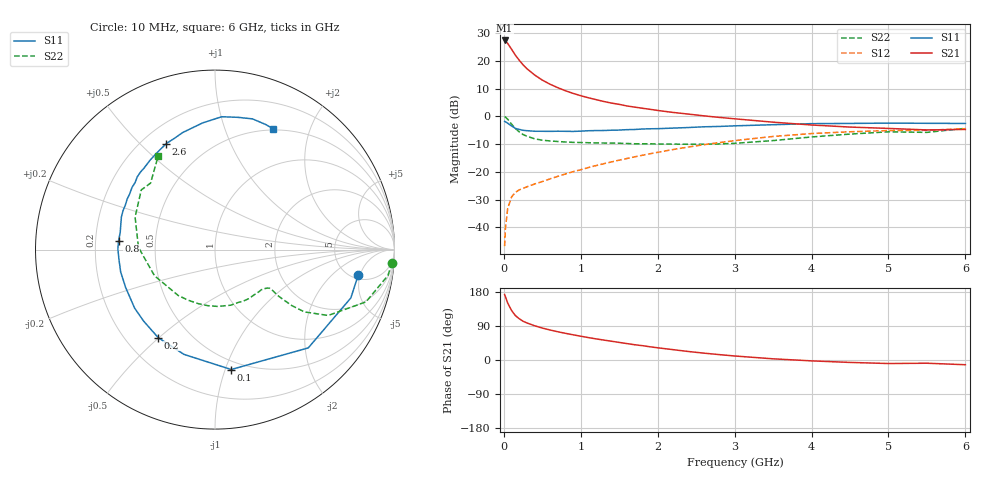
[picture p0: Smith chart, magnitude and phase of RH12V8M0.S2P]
! SIEMENS Small Signal Semiconductors
! BFR106
! Si NPN RF Bipolar Junction Transistor in SOT23
! VCE = 12 V  IC = 8 mA
! Common Emitter S-Parameters:  August  1996
# GHz  S  MA  R  50
!  f  S11  S21  S12  S22
! GHz  MAG  ANG  MAG  ANG  MAG  ANG  MAG  ANG
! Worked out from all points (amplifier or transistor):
!   36 points, 10 MHz to 6 GHz, reference 50 ohm
!   highest |S21| = 27.4 dB at 10 MHz (marker M1)
!   |S21| within 3 dB of that: start of sweep to 96.69 MHz
!   unconditionally stable (mu >= 1): 544.5 MHz to 1.88 GHz; 5.284 GHz to end of sweep
!   at 250 MHz: K = 0.63, MSG = 22.2 dB, |S12| = -25.9 dB
!   at 1.4 GHz: K = 1.11, MAG = 8.6 dB, |S12| = -16.4 dB
!   at 6 GHz: K = 1.01, MAG = -0.7 dB, |S12| = -4.4 dB
!   S11 on the Smith chart (normalised r, x): 10 MHz: 5.72, -4.65; 100 MHz: 0.43, -1.05; 200 MHz: 0.33, -0.50; 800 MHz: 0.30, +0.04; 2.6 GHz: 0.29, +0.60; 6 GHz: 0.48, +1.48
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0.01  0.8109 -9.9  23.36 172.7  0.0046 86.2  0.9878 -4.2
0.02  0.8033 -19.6  22.91 167.4  0.0095 80.4  0.9746 -8.5
0.05  0.755 -46.5  20.64 150.3  0.022 67.3  0.8902 -19.1
0.1  0.6741 -82.3  16.28 130.8  0.0353 54.8  0.7294 -30.2
0.15  0.6089 -106.5  12.68 117.2  0.0429 48.0  0.6065 -34.9
0.2  0.5838 -122.8  10.3 108.9  0.0475 46.3  0.5277 -36.1
0.25  0.5629 -134.9  8.496 102.3  0.0508 45.4  0.472 -36.2
0.3  0.5539 -144.0  7.235 97.8  0.0539 46.2  0.4391 -36.2
0.4  0.5407 -157.2  5.581 90.4  0.0607 49.1  0.3954 -35.4
0.5  0.5401 -166.7  4.513 84.3  0.0671 51.8  0.3729 -35.3
0.6  0.538 -174.3  3.806 79.2  0.075 54.8  0.362 -36.3
0.8  0.5396 174.7  2.902 70.4  0.0917 58.7  0.3461 -39.4
1.1  0.5524 160.7  2.166 59.1  0.1201 62.5  0.336 -46.7
1.3  0.5577 153.6  1.857 52.6  0.1408 63.6  0.3319 -52.3
1.6  0.5777 143.2  1.544 43.3  0.1746 63.6  0.3258 -62.4
2.2  0.6163 125.8  1.18 27.3  0.2532 60.0  0.3172 -86.9
2.6  0.6502 114.7  1.024 18.1  0.3092 55.3  0.3153 -106.8
3.5  0.7091 95.6  0.788 3.1  0.4357 41.1  0.3671 -156.5
4.5  0.748 80.1  0.643 -6.4  0.5293 22.4  0.4806 157.9
5  0.7577 74.0  0.608 -9.3  0.5558 14.1  0.5284 141.0
5.5  0.7519 67.8  0.571 -8.5  0.5632 9.6  0.5159 134.1
6  0.7471 64.4  0.583 -12.5  0.6013 1.5  0.6106 121.2
